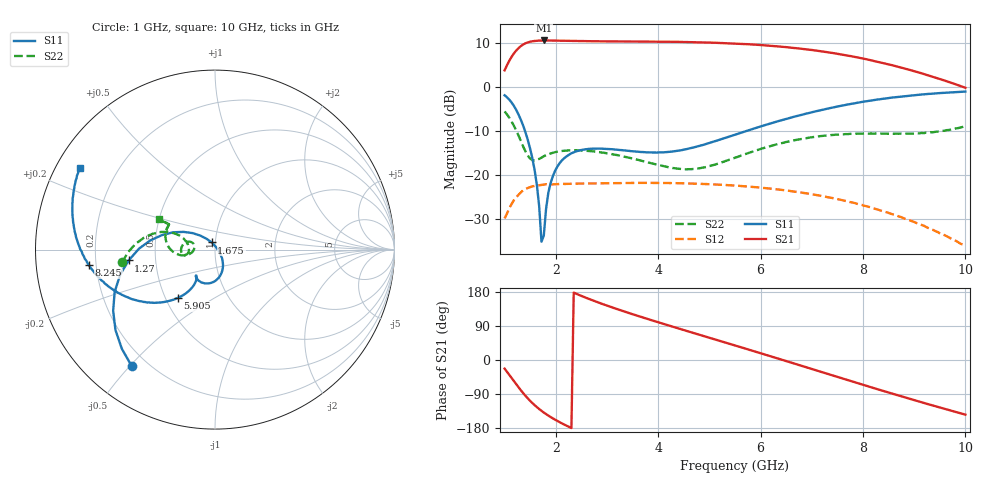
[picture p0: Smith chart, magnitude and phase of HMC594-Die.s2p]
! Analog Devices, Inc.
! Device:  HMC594-Die
! Description:  GaAs pHEMT MMIC LOW NOISE AMPLIFIER, 2-4 GHz
! Conditions:  Vdd = 6.0 V
!  Vgg = -0.8 V
!  Idd = 100 mA
!  Operating Temperature = +25C
! Engineering Evaluation unit (SN3) measured on PCB
! Measurements are referenced to PCB coaxial connectors with the exception of S21a(dB), for which the THRU CAL loss has been de-embedded.
! Freq(GHz)	S11a(dB)	S11p(deg)	S21a(dB)	S21p(deg)	S12a(dB)	S12p(deg)	S22a(dB)	S22p(deg)
# GHz S DB R 50
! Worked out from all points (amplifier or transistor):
!   201 points, 1 GHz to 10 GHz, reference 50 ohm
!   highest |S21| = 10.5 dB at 1.765 GHz (marker M1)
!   |S21| within 3 dB of that: 1.179 GHz to 7.483 GHz (6.304 GHz wide, 146 % of centre)
!   unconditionally stable (mu >= 1): start of sweep to end of sweep
!   at 2.485 GHz: K = 1.94, MAG = 10.6 dB, |S12| = -22.0 dB
!   at 5.5 GHz: K = 2.06, MAG = 10.3 dB, |S12| = -22.5 dB
!   at 10 GHz: K = 6.64, MAG = 6.8 dB, |S12| = -36.3 dB
!   S11 on the Smith chart (normalised r, x): 1 GHz: 0.14, -0.51; 1.27 GHz: 0.35, -0.05; 1.675 GHz: 0.96, +0.08; 5.905 GHz: 0.58, -0.35; 8.245 GHz: 0.17, -0.06; 10 GHz: 0.07, +0.28
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1  -1.96 -125.6  3.72 -22.8  -29.99 -130.2  -5.63 -172.2
1.135  -3.58 -149.0  6.77 -47.3  -26.72 -158.6  -7.91 170.6
1.27  -6.29 -172.9  8.74 -71.8  -24.61 174.0  -11.06 159.3
1.45  -11.99 157.4  10.05 -101.0  -23.06 141.5  -15.64 164.8
1.675  -27.18 114.8  10.48 -129.3  -22.43 109.5  -16.43 -173.0
1.72  -35.27 78.8  10.49 -134.1  -22.36 103.8  -16.15 -171.2
1.765  -33.93 -13.6  10.52 -138.6  -22.29 99.3  -15.83 -170.2
1.855  -24.05 -50.9  10.50 -146.8  -22.29 90.4  -15.38 -169.7
1.99  -19.04 -67.0  10.48 -157.8  -22.19 78.2  -14.89 -171.2
2.53  -14.34 -101.1  10.36 167.4  -22.04 41.4  -14.53 177.3
3.25  -14.41 -122.5  10.30 131.9  -21.91 5.9  -15.70 165.1
4.015  -14.96 -125.7  10.24 98.9  -21.90 -24.3  -17.85 163.8
4.735  -13.70 -121.2  10.11 69.4  -22.08 -49.8  -18.68 178.7
5.5  -10.92 -123.1  9.81 38.3  -22.51 -75.2  -16.17 -169.2
5.905  -9.40 -127.5  9.55 21.7  -22.89 -88.4  -14.54 -170.1
6.445  -7.52 -135.6  9.06 -0.6  -23.53 -105.5  -12.76 -176.3
7.03  -5.74 -146.6  8.30 -25.0  -24.54 -123.5  -11.47 174.1
7.57  -4.37 -157.9  7.35 -47.6  -25.76 -139.5  -10.86 164.8
8.245  -3.00 -172.9  5.78 -75.5  -27.81 -158.1  -10.65 155.6
8.514999  -2.58 -179.3  5.04 -86.6  -28.78 -164.8  -10.72 153.2
9.235001  -1.70 165.0  2.72 -115.2  -31.94 -179.5  -10.45 151.2
10  -1.11 149.0  -0.25 -144.2  -36.29 173.6  -9.01 151.3
